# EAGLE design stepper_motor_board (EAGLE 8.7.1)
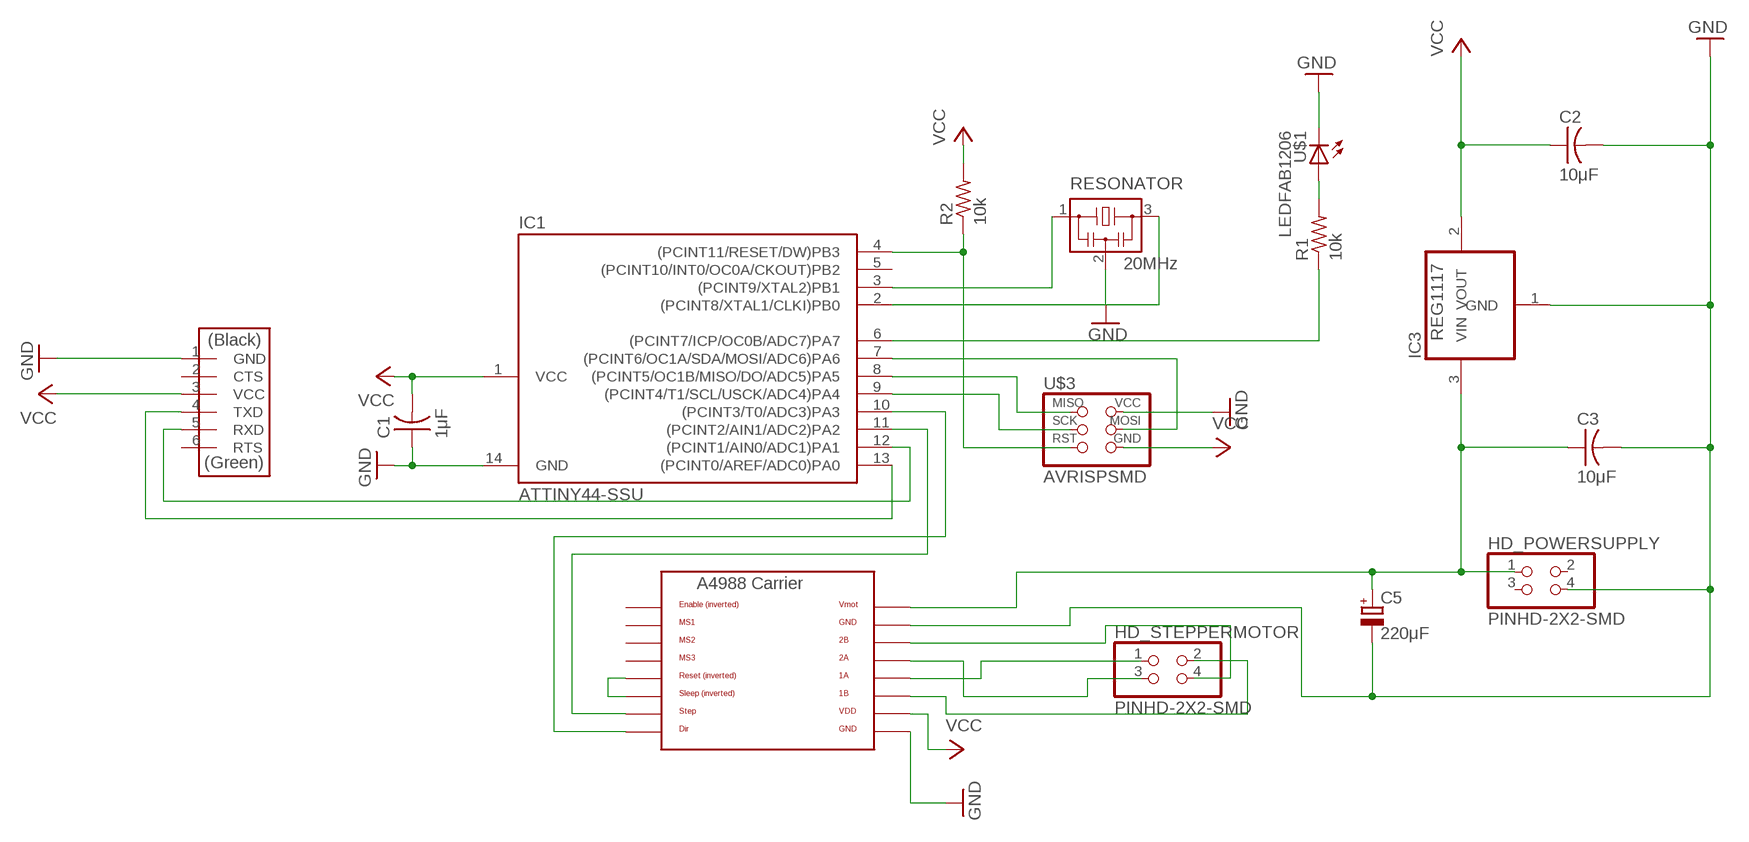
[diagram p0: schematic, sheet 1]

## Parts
C1  1μF  CAP-US1206FAB  [C1206FAB]
C2  10μF  CAP-US1206FAB  [C1206FAB]
C3  10μF  CAP-US1206FAB  [C1206FAB]
C5  220μF  CPOL-EUE5-10.5  [E5-10,5]
HD_POWERSUPPLY  PINHD-2X2-SMD  [2X02SMD]
HD_STEPPERMOTOR  PINHD-2X2-SMD  [2X02SMD]
IC1  ATTINY44-SSU  [SOIC14]
IC3  REG1117  [SOT223]
R1  10k  RES-US1206FAB  [R1206FAB]
R2  10k  RES-US1206FAB  [R1206FAB]
RESONATOR  20MHz  RESONATOR  [EFOBM]
U$1  LEDFAB1206  [LED1206FAB]
U$2  FTDI-SMD-HEADER  [1X06SMD]
U$3  AVRISPSMD  [2X03SMD]
U$5  A4983CARRIER  [A4988BREAKOUT]

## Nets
GND: C1.1 C2.2 C3.2 C5.- HD_POWERSUPPLY.4 IC1.14(GND) IC3.1(GND) RESONATOR.2 U$1.2(C) U$2.1(GND) U$3.2(VCC) U$5.GND U$5.GND@0(GND)
N$1: IC1.8((PCINT5/OC1B/MISO/DO/ADC5)PA5) U$3.1(MISO)
N$2: IC1.7((PCINT6/OC1A/SDA/MOSI/ADC6)PA6) U$3.4(MOSI)
N$3: IC1.9((PCINT4/T1/SCL/USCK/ADC4)PA4) U$3.3(SCK)
N$4: IC1.4((PCINT11/RESET/DW)PB3) R2.1 U$3.5(RST)
N$5: IC1.3((PCINT9/XTAL2)PB1) RESONATOR.1
N$6: IC1.2((PCINT8/XTAL1/CLKI)PB0) RESONATOR.3
N$7: HD_STEPPERMOTOR.1 U$5.1A
N$8: HD_STEPPERMOTOR.3 U$5.2A
N$9: HD_STEPPERMOTOR.4 U$5.2B
N$10: HD_STEPPERMOTOR.2 U$5.1B
N$11: U$5.RST U$5.SLP(SLEEP)
N$12: IC1.11((PCINT2/AIN1/ADC2)PA2) U$5.STEP
N$13: IC1.10((PCINT3/T0/ADC3)PA3) U$5.DIR
N$14: C3.1 C5.+ HD_POWERSUPPLY.1 IC3.3(VIN) U$5.VMOT
N$18: R1.2 U$1.1(A)
N$19: IC1.6((PCINT7/ICP/OC0B/ADC7)PA7) R1.1
N$20: IC1.13((PCINT0/AREF/ADC0)PA0) U$2.4(TXD)
N$21: IC1.12((PCINT1/AIN0/ADC1)PA1) U$2.5(RXD)
VCC: C1.2 C2.1 IC1.1(VCC) IC3.2(VOUT) R2.2 U$2.3(VCC) U$3.6(GND) U$5.VDD
Unconnected: HD_POWERSUPPLY.2 HD_POWERSUPPLY.3 IC1.5((PCINT10/INT0/OC0A/CKOUT)PB2) U$2.2(CTS) U$2.6(RTS) U$5.EN U$5.MS1 U$5.MS2 U$5.MS3

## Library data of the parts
C1-C3 = fab:CAP-US
C5 = rcl:CPOL-EU: POLARIZED CAPACITOR, European symbol; SPICEPREFIX: C
HD_POWERSUPPLY HD_STEPPERMOTOR = fab:PINHD-2X2-SMD
IC1 = fab:ATTINY44
IC3 = burr-brown:REG1117: 800mA and 1A Low Dropout (LDO) Positive Regulator 1.8V, 2.5V, 2.85V, 3.3V, 5V, and Adj; MPN: REG1117; OC_FARNELL: 1097566; OC_NEWARK: 14P6981
R1 R2 = fab:RES-US: Resistor (US Symbol)
RESONATOR = fab:RESONATOR
U$1 = fab:LED: LED
U$2 = fab:FTDI-SMD-HEADER
U$3 = fab:AVRISP
U$5 = RepRapjr:A4983CARRIER

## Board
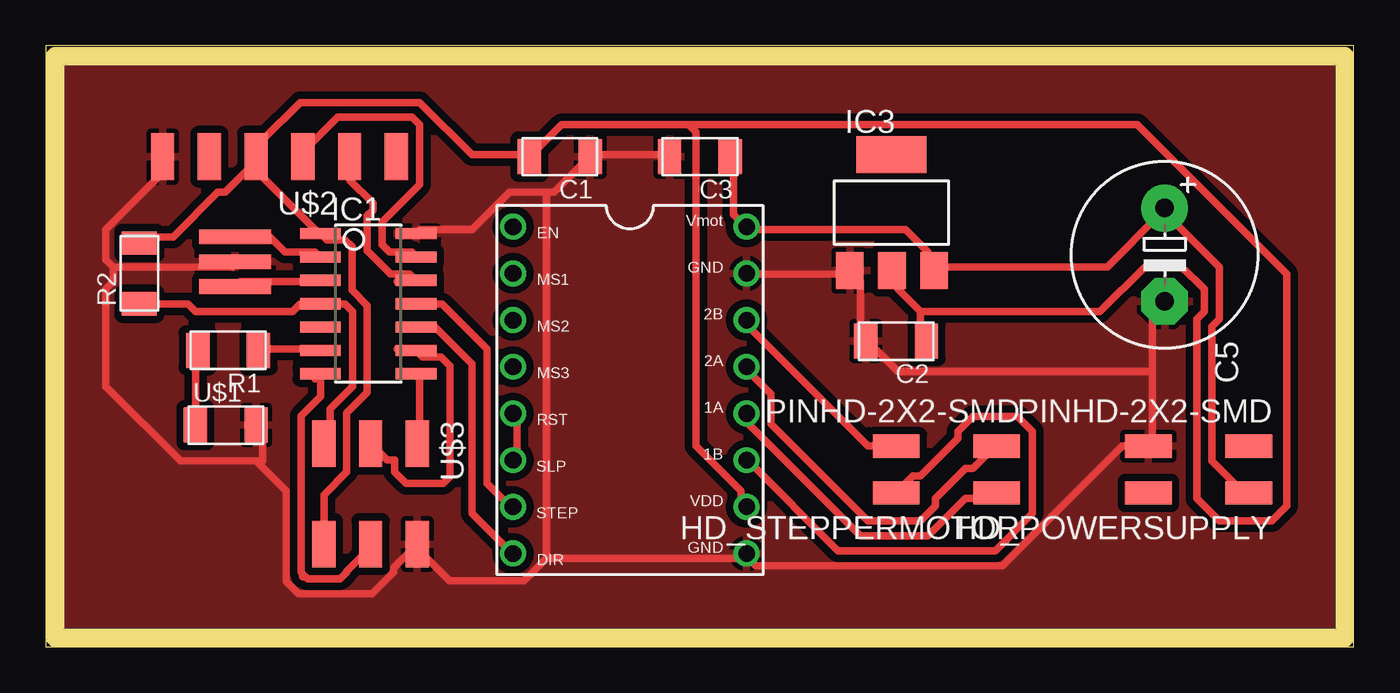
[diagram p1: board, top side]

Size 71.1 x 32.69 mm. Coordinates in mm from the lower left corner, seen from the top.
Outline: 0,0 71.1,0 71.1,32.69 0,32.69 0,0
Copper layers (1*16): Top 0.035mm / dielectric 1.5mm / Bottom 0.035mm
Design rules "default *": minimum track width 16mil, minimum drill 0.35mm, track to track 16mil, track to pad 16mil, pad to pad 16mil, via to via 16mil, smd to smd 16mil, copper to edge 40mil, drill to drill 16mil, minimum pad ring 10mil, minimum via ring 8mil, stop-mask expansion 4mil, vias tented up to drill 0mil, thermal gap 10mil
Milling: 4 lines

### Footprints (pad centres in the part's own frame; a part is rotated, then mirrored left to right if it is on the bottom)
C1206FAB = smd 1.27 x 1.905: 1 -1.651,0; 2 1.651,0
E5-10,5 = drill 1.016 pad 2.54: + -2.54,0 | drill 1.016 pad 2.54 octagon: - 2.54,0
2X02SMD = smd 2.54 x 1.27: 1 -2.54,1.27; 2 2.92,1.27; 3 -2.54,-1.27; 4 2.92,-1.27
SOIC14 = smd 0.61 x 2.21: 1 -3.81,-2.603; 2 -2.54,-2.603; 3 -1.27,-2.603; 4 0,-2.603; 5 1.27,-2.603; 6 2.54,-2.603; 7 3.81,-2.603; 8 3.81,2.603; 9 2.54,2.603; 10 1.27,2.603; 11 0,2.603; 12 -1.27,2.603; 13 -2.54,2.603; 14 -3.81,2.603
SOT223 = smd 1.499 x 2.007: 1 -2.261,-3.15; 2 0.025,-3.15; 3 2.311,-3.15 | smd 3.81 x 2.007: 4 0,3.15
R1206FAB = smd 1.27 x 1.905: 1 -1.651,0; 2 1.651,0
EFOBM = smd 0.8 x 3.9: 1 -1.35,0; 2 0,0; 3 1.35,0
LED1206FAB = smd 1.27 x 1.905: 1 -1.651,0; 2 1.651,0
1X06SMD = smd 2.54 x 1.27: 1 0,6.35; 2 0,3.81; 3 0,1.27; 4 0,-1.27; 5 0,-3.81; 6 0,-6.35
2X03SMD = smd 2.54 x 1.27: 1 -2.54,2.54; 2 2.92,2.54; 3 -2.54,0; 4 2.92,0; 5 -2.54,-2.54; 6 2.92,-2.54
A4988BREAKOUT = drill 0.9: 1A 8.89,1.27; 1B 11.43,1.27; 2A 6.35,1.27; 2B 3.81,1.27; DIR 16.51,-11.43; EN -1.27,-11.43; GND 16.51,1.27; GND@0 1.27,1.27; MS1 1.27,-11.43; MS2 3.81,-11.43; MS3 6.35,-11.43; RST 8.89,-11.43; SLP 11.43,-11.43; STEP 13.97,-11.43; VDD 13.97,1.27; VMOT -1.27,1.27

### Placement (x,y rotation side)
C1  27.94,26.67 180 top
C2  46.23,16.64 180 top
C3  35.56,26.67 180 top
C5  60.83,21.34 270 top
HD_POWERSUPPLY  62.87,9.65 180 top
HD_STEPPERMOTOR  49.15,9.65 180 top
IC1  17.53,18.67 270 top
IC3  45.97,23.62 0 top
R1  9.91,16.13 180 top
R2  5.08,20.32 90 top
RESONATOR  10.29,20.95 90 top
U$1  9.78,12.06 0 top
U$2  12.7,26.67 90 top
U$3  17.65,8.51 270 top
U$5  36.83,21.59 270 top

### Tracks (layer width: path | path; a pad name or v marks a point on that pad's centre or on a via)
GND
  Top 0.406: U$5.GND@0 38.2,20.27 43.48,20.27 IC3.1 43.89,20.27 44.3,19.86 44.3,17.02 C2.2 44.7,16.61 46.33,14.99 60.15,14.99 | 60.15,14.99 60.15,18.24 60.55,18.64 C5.- | 60.15,14.99 60.15,10.92 HD_POWERSUPPLY.4 58.52,10.92 52.02,4.42 38.61,4.42 38.2,4.83 U$5.GND 37.8,4.83 27.23,4.83 | C3.2 33.73,26.77 29.67,26.77 C1.1 29.26,26.36 27.64,24.74 27.23,24.74 | 27.23,24.74 25.2,24.74 23.16,22.71 20.32,22.71 IC1.14 | 3.66,20.68 3.25,21.08 3.25,22.71 6.1,25.55 6.1,26.36 U$2.1 | 3.66,20.68 10.16,20.68 RESONATOR.2 | U$1.2 11.79,11.73 11.79,10.11 11.43,10.11 | 27.23,4.83 26.01,3.61 21.95,3.61 20.32,5.23 U$3.2 18.9,4.29 18.9,4.07 17.73,2.9 13.73,2.9 13.06,3.58 13.06,8.48 11.43,10.11 | 3.66,20.68 3.66,19.86 3.25,19.46 3.25,14.17 7.32,10.11 11.43,10.11 | 27.23,4.83 27.23,24.74
  pour Top: 0,33.02 71.12,33.02 71.12,0 0,0
N$1
  Top 0.406: IC1.8 20.32,14.58 20.32,11.33 U$3.1
N$2
  Top 0.406: 14.63,14.58 IC1.7 14.92,13.63 13.87,12.57 13.87,4.07 13.97,3.96 13.97,3.81 14.12,3.81 14.22,3.71 16,3.71 16.36,4.07 16.36,4.12 17.88,5.64 U$3.4
N$3
  Top 0.406: 19.1,16.2 19.91,16.2 IC1.9 20.48,15.77 21.49,15.77 21.97,15.29 21.97,9.27 21.59,8.89 19.59,8.89 18.95,9.53 18.95,10.16 18.54,10.16 U$3.3 17.88,11.33
N$4
  Top 0.406: R2.1 5.28,18.64 7.72,18.64 8.13,18.24 13.41,18.24 13.82,18.64 14.63,18.64 IC1.4 15.04,18.64 16.26,18.64 16.66,18.24 16.66,14.17 15.44,12.95 15.44,11.33 U$3.5
N$5
  Top 0.406: IC1.3 14.63,19.86 10.57,19.86 RESONATOR.1
N$6
  Top 0.406: IC1.2 14.63,21.49 13.01,21.49 12.19,22.3 10.57,22.3 RESONATOR.3
N$7
  Top 0.406: HD_STEPPERMOTOR.1 51.61,8.08 49.99,8.08 47.95,6.04 44.3,6.04 37.8,12.55 U$5.1A
N$8
  Top 0.406: HD_STEPPERMOTOR.3 51.61,10.92 50.39,9.7 49.99,9.7 48.36,8.08 48.36,7.67 47.55,6.86 44.7,6.86 39.42,12.14 39.42,13.77 38.2,14.99 U$5.2A
N$9
  Top 0.406: HD_STEPPERMOTOR.4 44.7,10.92 38.2,17.42 U$5.2B
N$10
  Top 0.406: HD_STEPPERMOTOR.2 46.33,8.48 47.14,9.3 47.55,9.3 49.58,11.33 49.58,11.73 50.39,12.55 52.83,12.55 53.65,11.73 53.65,7.26 51.61,5.23 43.08,5.23 38.2,10.11 U$5.1B
N$11
  Top 0.406: U$5.SLP 25.6,10.52 25.6,12.55 U$5.RST
N$12
  Top 0.406: IC1.11 20.32,18.64 21.54,18.64 23.98,16.2 23.98,8.89 25.2,7.67 U$5.STEP
N$13
  Top 0.406: IC1.10 20.32,17.42 21.13,17.42 23.16,15.39 23.16,7.26 25.2,5.23 U$5.DIR
N$14
  Top 0.406: C3.1 37.39,26.36 37.39,23.52 37.8,23.11 U$5.VMOT 38.2,22.71 46.74,22.71 47.95,21.49 47.95,20.68 IC3.3 48.36,20.68 57.71,20.68 60.55,23.52 C5.+ 60.96,23.52 63.8,20.68 63.8,17.83 63.4,17.42 63.4,10.11 65.02,8.48 HD_POWERSUPPLY.1
N$18
  Top 0.406: U$1.1 8.13,15.8 R1.2
N$19
  Top 0.406: R1.1 11.79,16.2 14.63,16.2 IC1.6
N$20
  Top 0.406: IC1.13 19.91,21.49 18.69,21.49 18.29,21.89 18.29,23.11 20.32,25.15 20.32,28.4 19.91,28.8 15.85,28.8 13.82,26.77 U$2.4
N$21
  Top 0.406: 19.1,19.86 19.91,19.86 IC1.12 19.77,20.3 18.74,20.3 17.48,21.56 17.48,23.45 17.78,23.75 17.78,24.13 16.51,25.4 U$2.5 16.66,26.36
VCC
  Top 0.406: 47.55,18.24 47.55,17.02 C2.1 | 47.55,18.24 46.33,19.46 46.33,20.27 IC3.2 | R2.2 5.28,22.3 6.91,22.3 9.35,24.74 9.75,24.74 11.38,26.36 U$2.3 | U$2.3 11.79,26.77 11.79,27.58 13.82,29.62 20.32,29.62 23.16,26.77 26.01,26.77 C1.2 26.42,26.77 28.04,28.4 34.95,28.4 | U$2.3 11.79,26.36 11.79,25.55 14.63,22.71 IC1.1 15.28,22.12 16.28,22.12 16.64,21.77 16.64,19.41 17.48,18.57 17.48,13.84 16.36,12.72 16.36,9.53 15.11,8.28 U$3.6 | 34.95,28.4 35.36,27.99 35.36,10.92 37.8,8.48 37.8,7.67 U$5.VDD | 47.55,18.24 57.3,18.24 59.74,20.68 61.77,20.68 62.99,19.46 62.99,18.24 62.59,17.83 62.59,8.08 63.8,6.86 66.65,6.86 67.46,7.67 67.46,20.27 59.33,28.4 34.95,28.4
